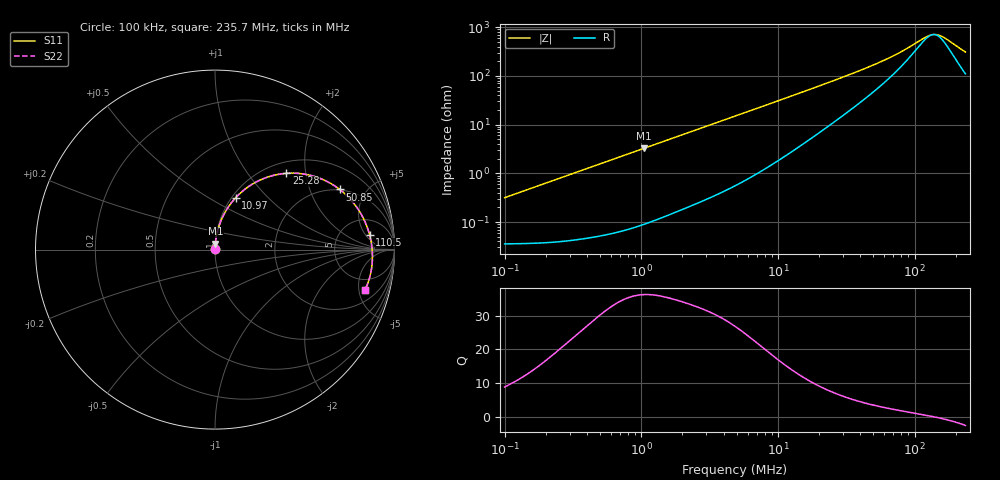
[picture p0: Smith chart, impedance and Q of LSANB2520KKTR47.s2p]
! LSANB2520KKTR47  S-PARAMETER MODEL  ( General Type )
! Model Generated by TAIYO YUDEN Corporation (http://www.ty-top.com)
! Version 2.0
! TAIYO YUDEN Control No. 20210629
! Copyright(c) 2013 TAIYO YUDEN CO.,LTD. All Rights Reserved.
! Product Description (link to TY-COMPAS)
! https://ds.yuden.co.jp/TYCOMPAS/or/detail?pn=LSANB2520KKTR47M&u=M
! Products Name : Inductors
! Characteristics :
!  Inductance : 0.47 uH , SRF(min) : -Hz , DC Resistance(max) : 0.046 Ohm
!  Rated Current : Saturation :3900 mA , Temp Rise : 3200 mA (40 degC)
!  Case Size : 2.5 x 2.0 / 0.098 x 0.079 [mm/inch] , Thickness : 1 / 0.039 [mm/inch]
!  (Conditions: Temperature = 25 degC , DC Bias Current/Voltage = 0A / 0V)
! External Node Assignments :
!  1  o---GGG---o  2
! GND o---------o GND
! Frequency Range : 0.1MHz  -  235.669543MHz  [ 402 STEP ]
# MHz S RI R 50
! Freq[MHz].  S11 Real  S11 Imag  S21 Real  S21 Imag  S12 Real  S12 Imag  S22 Real  S22 Imag
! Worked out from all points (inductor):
!   401 points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, 100 kHz to 235.7 MHz, reference 50 ohm
!   read as one part in series: L = 499 nH near 104 kHz
!   highest Q = 36.3 at 1.047 MHz (marker M1), where L = 495 nH
!   self-resonance near 136.9 MHz
!   S11 on the Smith chart (normalised r, x): 100 kHz: 1.00, +0.01; 10.97 MHz: 1.04, +0.67; 25.28 MHz: 1.22, +1.56; 50.85 MHz: 1.97, +3.27; 110.5 MHz: 10, +6; 235.7 MHz: 3.20, -5.77
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0.1  0.000365 0.00313  0.9996 -0.00313  0.9996 -0.00313  0.000365 0.00313
0.367165  0.000579 0.0115  0.9994 -0.0115  0.9994 -0.0115  0.000579 0.0115
1.047422  0.00195 0.0325  0.998 -0.0325  0.998 -0.0325  0.00195 0.0325
1.348099  0.0029 0.0416  0.9971 -0.0416  0.9971 -0.0416  0.0029 0.0416
2.711621  0.00942 0.0824  0.9906 -0.0824  0.9906 -0.0824  0.00942 0.0824
4.854581  0.0267 0.1437  0.9733 -0.1437  0.9733 -0.1437  0.0267 0.1437
7.586809  0.0604 0.2154  0.9396 -0.2154  0.9396 -0.2154  0.0604 0.2154
10.97093  0.1161 0.2901  0.8839 -0.2901  0.8839 -0.2901  0.1161 0.2901
14.12029  0.1768 0.3439  0.8232 -0.3439  0.8232 -0.3439  0.1768 0.3439
17.8243  0.2522 0.3879  0.7478 -0.3879  0.7478 -0.3879  0.2522 0.3879
25.27937  0.3968 0.4249  0.6032 -0.4249  0.6032 -0.4249  0.3968 0.4249
35.16326  0.5475 0.4096  0.4525 -0.4096  0.4525 -0.4096  0.5475 0.4096
50.84796  0.6953 0.3349  0.3047 -0.3349  0.3047 -0.3349  0.6953 0.3349
65.44454  0.7712 0.2607  0.2288 -0.2607  0.2288 -0.2607  0.7712 0.2607
84.23125  0.8252 0.1771  0.1748 -0.1771  0.1748 -0.1771  0.8252 0.1771
110.536  0.8617 0.0807  0.1383 -0.0807  0.1383 -0.0807  0.8617 0.0807
129.107  0.8731 0.0226  0.1269 -0.0226  0.1269 -0.0226  0.8731 0.0226
139.5317  0.8762 -0.00735  0.1238 0.00735  0.1238 0.00735  0.8762 -0.00735
147.899  0.8772 -0.0303  0.1228 0.0303  0.1228 0.0303  0.8772 -0.0303
166.1689  0.8756 -0.0775  0.1244 0.0775  0.1244 0.0775  0.8756 -0.0775
218.0622  0.8494 -0.193  0.1506 0.193  0.1506 0.193  0.8494 -0.193
235.6695  0.835 -0.2266  0.165 0.2266  0.165 0.2266  0.835 -0.2266
